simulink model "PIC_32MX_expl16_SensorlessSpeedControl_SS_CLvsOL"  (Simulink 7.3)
settings: Solver=FixedStepDiscrete  StartTime=0.0  StopTime=10.0  FixedStep=.002  RelTol=1e-3
InitFcn:
  | Synthese_controleurPicooz_StateSpace_Integrateur;
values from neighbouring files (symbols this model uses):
  Az = [0.8544 0.9806]    [Synthese_controleurPicooz_StateSpace_Integrateur.m]
  Bz = [-0.0207 0.0659]'    [Synthese_controleurPicooz_StateSpace_Integrateur.m]
  Cz = [-0.0319   -0.0107]    [Synthese_controleurPicooz_StateSpace_Integrateur.m]
undefined symbols (not defined in the file or in its folder): bits, Buffer, characters, contain, DiscIntNeverNeededParam, full, is, OC_HW, OCmax, PWM, Receive, Timer3, When
libraries: dsPICdrivers x8, simulink x1

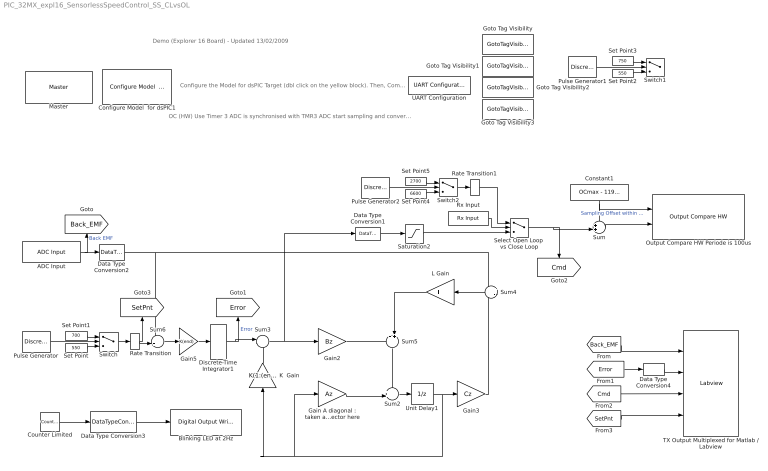
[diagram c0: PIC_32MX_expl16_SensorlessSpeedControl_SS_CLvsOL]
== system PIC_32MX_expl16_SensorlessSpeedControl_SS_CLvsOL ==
  note: Demo (Explorer 16 Board) - Updated 13/02/2009
  note: Configure the Model for dsPIC Target (dbl click on the yellow block). Then, Compile using the incremental build icon (second icon on right of the simulation mode (Normal))
  note: OC (HW) Use Timer 3 ADC is synchronised with TMR3 ADC start sampling and converting when TMR3 = OCmax (=PR3)
  ADC Input : dsPICdrivers/Peripheral I//O/ADC Input  Tag=dsPIC_ADC  Priority=5  ADC_TYPE=10 bits  ADC_MODE=Continuous sampling & get last channel value  NbrSampleStep=1  VoltRefpopup="AVdd  -  AVss"  OutFormatBitspopup=0000 00dd dddd dddd : Integer  InterruptPriority=6  ANCHANNELS=5  MaxName=ANmax = 1023  Rin=5e6  ADCS=29  SAMC=31  Temperature=25  DMAChannel=0  SampleTime=.002  Status="OK  |  Tsmp=4.844e-006 |  T/Channel=6.719e-006 |  Tall=6.719e-006"  SSRC=Timer3 (OC_HW PWM)
  Blinking LED at 2Hz : dsPICdrivers/Digital I//O/Digital Output Write  Tag=dsPIC_Digital_Output  Priority=5  PORT=A  Pin=[2]  Simultaneous=off  OrderingInOutPopup=None
  Configure Model  for dsPIC1 : dsPICdrivers/Simulink Configuration/Configure Model  for dsPIC
  Constant1 : Constant  Value=OCmax - 11970  OutDataTypeMode=uint16  OutDataType=sfix(16)  OutScaling=2^0  OutDataTypeStr=uint16
  Counter Limited : simulink/Sources/Counter Limited  SystemSampleTime=-1  uplimit=1  tsamp=.25
  Data Type Conversion1 : DataTypeConversion  OutDataTypeMode=uint16  OutDataType=sfix(16)  OutScaling=2^0  OutDataTypeStr=uint16
  Data Type Conversion2 : DataTypeConversion  OutDataTypeMode=double  OutDataType=sfix(16)  OutScaling=2^0  OutDataTypeStr=double
  Data Type Conversion3 : DataTypeConversion  OutDataTypeMode=boolean  OutDataType=sfix(16)  OutScaling=2^0  OutDataTypeStr=boolean
  Data Type Conversion4 : DataTypeConversion  OutDataTypeMode=uint16  OutDataType=sfix(16)  OutScaling=2^0  OutDataTypeStr=uint16  ConvertRealWorld=Stored Integer (SI)
  Discrete-Time Integrator1 : DiscreteIntegrator  gainval=1  SampleTime=.002  OutDataType=fixdt(1,32,20)  SaturateOnIntegerOverflow=on  LimitOutput=on  UpperSaturationLimit=400000  LowerSaturationLimit=-400000  ICPrevOutput=DiscIntNeverNeededParam  ICPrevScaledInput=DiscIntNeverNeededParam
  "Gain A diagonal : taken as a vector here" : Gain  Gain=Az  ParameterDataType=sfix(16)  ParameterScaling=2^0  OutDataType=sfix(16)  OutScaling=2^0
  Gain2 : Gain  Gain=Bz  Multiplication=Matrix(K*u)  ParameterDataType=sfix(16)  ParameterScaling=2^0  OutDataType=sfix(16)  OutScaling=2^0
  Gain3 : Gain  Gain=Cz  Multiplication=Matrix(K*u)  ParameterDataType=sfix(16)  ParameterScaling=2^0  OutDataType=sfix(16)  OutScaling=2^0
  Gain5 : Gain  Gain=K(end)  Multiplication=Matrix(K*u)  ParameterDataType=sfix(16)  ParameterScaling=2^0  OutDataType=sfix(16)  OutScaling=2^0
  Goto Tag Visibility{,1..3} (4 alike) : GotoTagVisibility
  K  Gain : Gain  Gain=K(1:(end-1))  Multiplication=Matrix(K*u)  ParameterDataType=sfix(16)  ParameterScaling=2^0  OutDataType=sfix(16)  OutScaling=2^0
  L Gain : Gain  Gain=L'  Multiplication=Matrix(K*u)  ParameterDataType=sfix(16)  ParameterScaling=2^0  OutDataType=sfix(16)  OutScaling=2^0
  Master : dsPICdrivers/Master  Tag=dsPIC_MASTER  Priority=1  TimeStepType=Timer1  picType=32MX460F512L  fcy=96000000  Quartz_33f=8e6  PLLActive_33f=on  fcyDesired_33f=96e6  tmr1="[8  23999  0]"  tmr1Info="Time Step : 0.002  ;   Error : 0%  PR1=23999"  tmr2345="[0  8  0  0]"  tmr2345cfg=[-1 -1 -1 -1]  IOautoConf=on  typePort="[ 0   0  10   0   0   0   0   0   0   0   0   0   0   0   0   0   0   0   0   0   0   8   0   0   0   0   0   0   0   0   0   0   0   0   0   0   0   0   0   0   0   0   0   0   0   0   0   0  24   0   0   0   0   0   0   0   0   0   0   0   0   0   0   0   0   0   0   0   0   0   0   0   0   0   0   0   0   0   0   0   0   0   0   0   4   5   0   0   0   0   0   0   0   0   0   0   0   0   0   0 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"  TRIS="[ 65531  65535  65535  65534  65535  65535  65535 ]"  ADPCFG=0  MasterBusyPort=None  MasterOverloadPort=None  FOSC=Quartz (XT - HS)  ClockSwitchMonitor=Both disabled  TempProtection_33f=TEMP_ON  FPBOR=<empty>  PWRT=disable  MCLR=<empty>  PowerSave=off  OverrideFcy=off  NewFcy=1e6  PR2345="[65535  11999  65535  65535]"
  Output Compare HW Periode is 100us : dsPICdrivers/Peripheral I//O/Output Compare HW  Tag=dsPIC_OC_HW_out  Priority=5  OC_Mode=PWM Time Set-Reset (glitch possible)  Timer=3  CHANNEL=[1 ]  Channel_UP_Down_Periode=[16]  PeriodeInput=off  MaxChannel=0.001  MaxName=' OCmax '  Precision=[13.5507]  Status=OK  SafeMarge=[0]  PortLetter=[68]  PortNumber=[0]  MaxValues=[11999]  NPORTS=2
  Pulse Generator : DiscretePulseGenerator  Amplitude=1  Period=4  PulseWidth=2  PhaseDelay=0  SampleTime=1
  Pulse Generator1 : DiscretePulseGenerator  Amplitude=1  Period=2  PulseWidth=1  PhaseDelay=0  SampleTime=1
  Pulse Generator2 : DiscretePulseGenerator  Amplitude=1  Period=4  PulseWidth=2  PhaseDelay=0  SampleTime=1
  Rate Transition : RateTransition
  Rate Transition1 : RateTransition
  Rx Input : dsPICdrivers/Serial PORT/Rx Input  Tag=dsPIC_RX  Priority=5  UART=2  SampleTime=-1  BlockingFctChk=off  OutputDefault=-1  IsPresentFlagChk=off
  Saturation2 : Saturate  UpperLimit=OCmax-500  LowerLimit=500  OutDataType=sfix(16)  OutScaling=2^0
  Select Open Loop  vs Close Loop : Switch  Criteria=u2 ~= 0  OutDataType=fixdt(1, 16)  OutScaling=2^0
  Set Point : Constant  Value=550  OutDataTypeMode=uint16  OutDataType=sfix(16)  OutScaling=2^0  OutDataTypeStr=uint16
  Set Point1 : Constant  Value=700  OutDataTypeMode=uint16  OutDataType=sfix(16)  OutScaling=2^0  OutDataTypeStr=uint16
  Set Point2 : Constant  Value=550  OutDataType=sfix(16)  OutScaling=2^0  OutDataTypeStr=Inherit: Inherit via back propagation
  Set Point3 : Constant  Value=750  OutDataType=sfix(16)  OutScaling=2^0  OutDataTypeStr=Inherit: Inherit via back propagation
  Set Point4 : Constant  Value=6600  OutDataTypeMode=uint16  OutDataType=sfix(16)  OutScaling=2^0  OutDataTypeStr=uint16
  Set Point5 : Constant  Value=2700  OutDataTypeMode=uint16  OutDataType=sfix(16)  OutScaling=2^0  OutDataTypeStr=uint16
  Sum : Sum  Inputs=++|  AccumDataTypeStr=int16  OutDataTypeMode=uint16  OutDataType=sfix(16)  OutScaling=2^0  OutDataTypeStr=uint16
  Sum2 : Sum  Inputs=++|  AccumDataTypeStr=double  OutDataType=sfix(16)  OutScaling=2^0
  Sum3 : Sum  Inputs=|--  OutDataType=sfix(16)  OutScaling=2^0
  Sum4 : Sum  Inputs=+-  OutDataType=sfix(16)  OutScaling=2^0
  Sum5 : Sum  Inputs=++|  OutDataType=sfix(16)  OutScaling=2^0
  Sum6 : Sum  Inputs=-+|  OutDataType=sfix(16)  OutScaling=2^0
  Switch : Switch  Criteria=u2 ~= 0  OutDataType=fixdt(1, 16)  OutScaling=2^0
  Switch1 : Switch  Criteria=u2 ~= 0  OutDataType=fixdt(1, 16)  OutScaling=2^0
  Switch2 : Switch  Criteria=u2 ~= 0  OutDataType=fixdt(1, 16)  OutScaling=2^0
  TX Output Multiplexed for Matlab / Labview : dsPICdrivers/Serial PORT/TX Output Multiplexed for Matlab // Labview  Tag=dsPIC_TX_Multiplexed  Priority=5  UART=2  CleverSpreadingChk=on  CleverSpreading=1  CHANNEL=[0:3]  CHANNELBLOCKED=[]  CHANNELBLOCKED_BITEWISE=0  Status=OK
  UART Configuration : dsPICdrivers/Serial PORT/UART Configuration  Tag=dsPIC_config_UART  Priority=2  UART=2  proposed_BAUD=115200  ALT_TX_RX=on  InterruptTxWhen=When Transmit Buffer is empty  TXInterruptPri=1  TxBufferSize=32  TXEN=on  InterruptRxWhen=When Receive Buffer is full (contain 4 characters)  RXInterruptPri=2  RxBufferSize=32  BAUD=115200  UxBRG=51  Info="UxBRG = 51   ||  Real Baud : 115385   ||  % error : 0.16026  ||  max 23.0769 Bytes / Step"  RealBaud=0
  Unit Delay1 : UnitDelay  X0=[0 0]  SampleTime=-1
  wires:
  Counter Limited/1 -> Data Type Conversion3/1
  Sum/1 -> Output Compare HW Periode is 100us/2
  Constant1/1 -> Output Compare HW Periode is 100us/1, Sum/1  "Sampling Offset within PWM"
  Data Type Conversion3/1 -> Blinking LED at 2Hz/1
  Sum2/1 -> Unit Delay1/1
  "Gain A diagonal : taken as a vector here"/1 -> Sum2/2
  Gain3/1 -> Sum4/2
  Sum3/1 -> Gain2/1, Data Type Conversion1/1
  Gain2/1 -> Sum5/1
  Sum6/1 -> Gain5/1
  Unit Delay1/1 -> "Gain A diagonal : taken as a vector here"/1, K  Gain/1, Gain3/1
  Sum5/1 -> Sum2/1
  K  Gain/1 -> Sum3/2
  Gain5/1 -> Discrete-Time Integrator1/1
  Discrete-Time Integrator1/1 -> Sum3/1, [Error]  "Error"
  Sum4/1 -> L Gain/1
  L Gain/1 -> Sum5/2
  Data Type Conversion1/1 -> Saturation2/1
  Data Type Conversion2/1 -> Sum6/1, Sum4/1
  ADC Input/1 -> Data Type Conversion2/1, [Back_EMF]  "Back EMF"
  [Back_EMF] -> TX Output Multiplexed for Matlab / Labview/1
  [Error] -> Data Type Conversion4/1
  [Cmd] -> TX Output Multiplexed for Matlab / Labview/3
  Data Type Conversion4/1 -> TX Output Multiplexed for Matlab / Labview/2
  Pulse Generator/1 -> Switch/2
  Set Point/1 -> Switch/3
  Set Point1/1 -> Switch/1
  Switch/1 -> Rate Transition/1
  Rate Transition/1 -> Sum6/2, [SetPnt]
  [SetPnt] -> TX Output Multiplexed for Matlab / Labview/4
  Pulse Generator1/1 -> Switch1/2
  Set Point2/1 -> Switch1/3
  Set Point3/1 -> Switch1/1
  Pulse Generator2/1 -> Switch2/2
  Set Point4/1 -> Switch2/3
  Set Point5/1 -> Switch2/1
  Saturation2/1 -> Select Open Loop  vs Close Loop/3
  Select Open Loop  vs Close Loop/1 -> Sum/2, [Cmd]
  Switch2/1 -> Rate Transition1/1
  Rx Input/1 -> Select Open Loop  vs Close Loop/2
  Rate Transition1/1 -> Select Open Loop  vs Close Loop/1
